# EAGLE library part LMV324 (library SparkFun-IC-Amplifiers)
IC LMV324 Quad Op Amp Jellybean quad op-amp Datasheet SparkFun Products SparkFun Sensor Kit (DEV-13754) SparkFun Inventor's Kit for Arduino 101 (KIT-13844) SparkFun Sound Detector (SEN-12642)
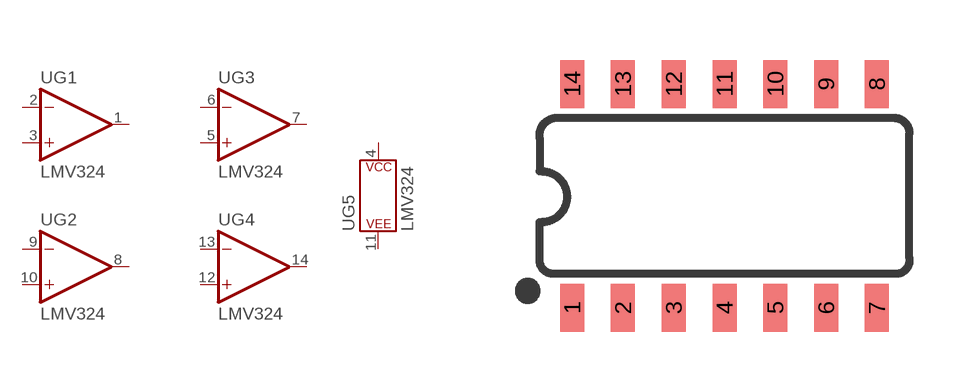
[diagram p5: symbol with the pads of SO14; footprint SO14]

Designator prefix U; gates G1=OP-AMP G2=OP-AMP G3=OP-AMP G4=OP-AMP G5=POWER_CONSORT

## LMV324 (PROD_ID: IC-08227; VALUE: LMV324)  [SO14]
1  G1:OUT  out
2  G1:-IN  in
3  G1:+IN  in
4  G5:P$V+
5  G3:+IN  in
6  G3:-IN  in
7  G3:OUT  out
8  G2:OUT  out
9  G2:-IN  in
10  G2:+IN  in
11  G5:P$V-
12  G4:+IN  in
13  G4:-IN  in
14  G4:OUT  out

## Footprint SO14 (pad centres in mm)
SOIC, 0.15 inch width
smd 0.6 x 1.2: 1 -3.175,-2.8; 2 -1.905,-2.8; 3 -0.635,-2.8; 4 0.635,-2.8; 5 1.905,-2.8; 6 3.175,-2.8; 7 4.445,-2.8; 8 4.445,2.8; 9 3.175,2.8; 10 1.905,2.8; 11 0.635,2.8; 12 -0.635,2.8; 13 -1.905,2.8; 14 -3.175,2.8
